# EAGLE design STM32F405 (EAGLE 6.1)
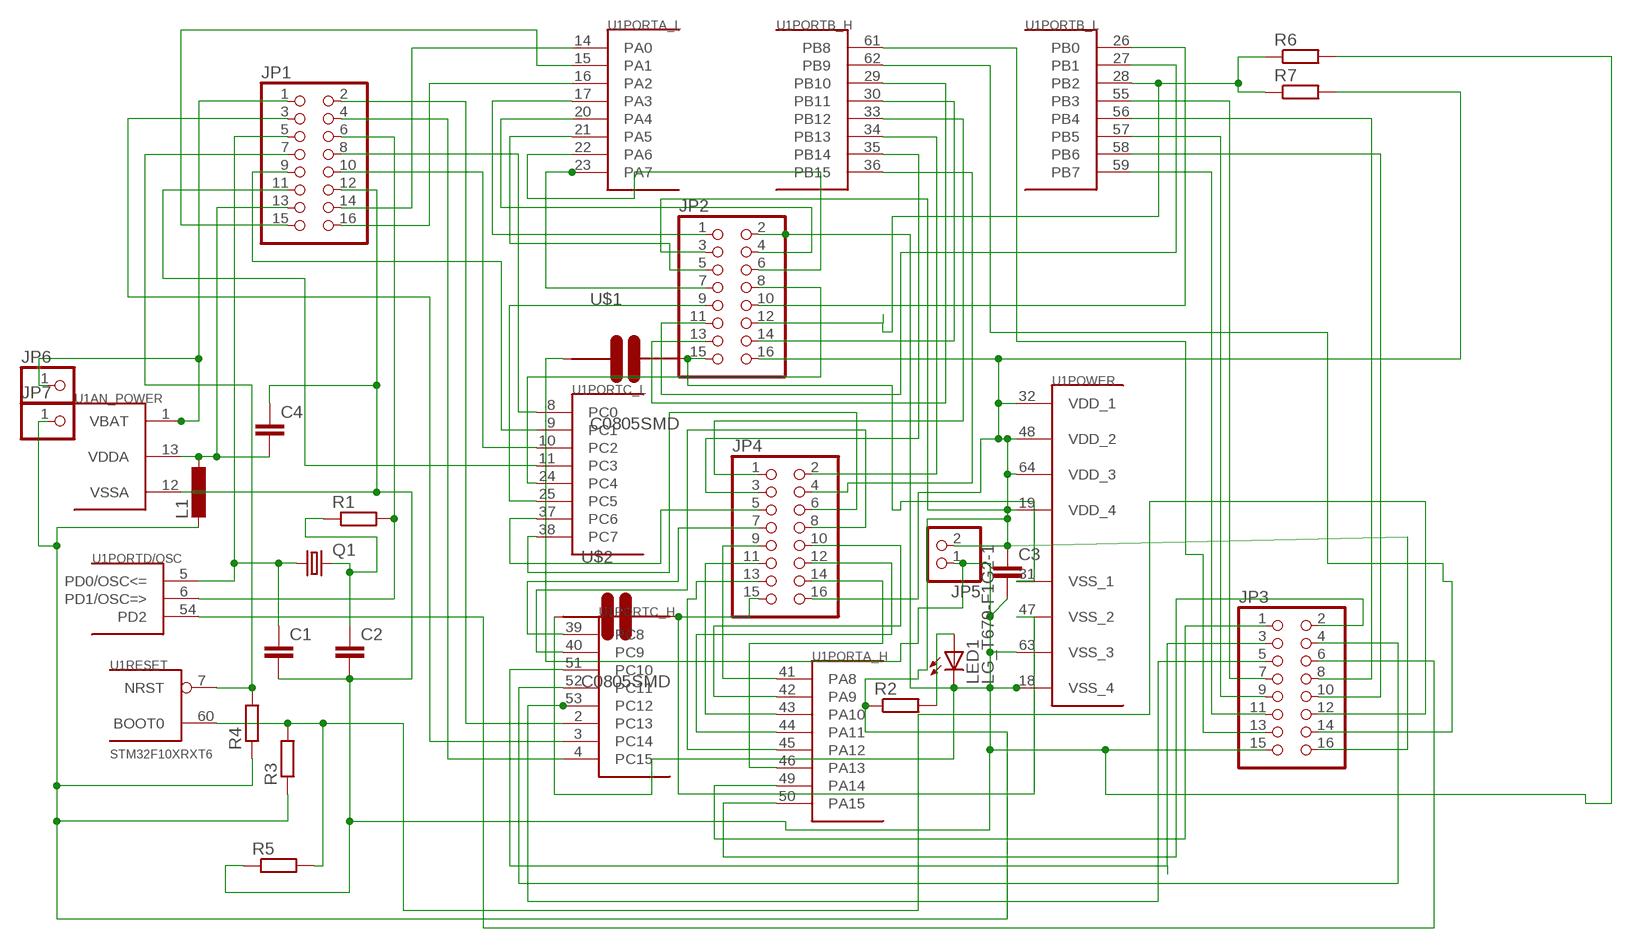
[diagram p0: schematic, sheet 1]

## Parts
C1  C-EUC0805  [C0805]
C2  C-EUC0805  [C0805]
C3  C-EUC1206  [C1206]
C4  C-EUC0805  [C0805]
JP1  PINHD-2X8  [2X08]
JP2  PINHD-2X8  [2X08]
JP3  PINHD-2X8  [2X08]
JP4  PINHD-2X8  [2X08]
JP5  PINHD-1X2  [1X02]
JP6  PINHD-1X1  [1X01]
JP7  PINHD-1X1  [1X01]
L1  L-EUL1812  [L1812]
LED1  LG_T679-F1G2-1  [PLCC2]
Q1  CRYSTALHC49S  [HC49/S]
R1  R-EU_R0805  [R0805]
R2  R-EU_R0805  [R0805]
R3  R-EU_R0805  [R0805]
R4  R-EU_R0805  [R0805]
R5  R-EU_R0805  [R0805]
R6  R-EU_M0805  [M0805]
R7  R-EU_M0805  [M0805]
U1  STM32F10XRXT6  [TQFP64]
U$1  C0805SMD  [C0805]
U$2  C0805SMD  [C0805]

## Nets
N$1: JP2.8 U1.24(PORTC_L:PC4)
N$2: C3.1 JP2.3 JP2.16 JP3.16 JP4.16 JP5.2 JP7.1 L1.2 R2.1 R3.1 R4.1 R7.2 U1.19(POWER:VDD_4) U1.32(POWER:VDD_1) U1.48(POWER:VDD_2) U1.64(POWER:VDD_3)
N$3: C4.2 JP1.13 L1.1 U1.13(AN_POWER:VDDA)
N$6: JP1.6 R1.2 U1.6(PORTD/OSC:PD1/OSC=>)
N$7: JP1.7 R4.2 U1.7(RESET:NRST)
N$8: JP1.14 U1.14(PORTA_L:PA0)
N$9: JP1.16 U1.16(PORTA_L:PA2)
N$10: JP1.15 U1.15(PORTA_L:PA1)
N$11: JP1.8 U1.8(PORTC_L:PC0)
N$12: JP1.9 U1.9(PORTC_L:PC1)
N$13: JP1.10 U1.10(PORTC_L:PC2)
N$14: JP1.11 U1.11(PORTC_L:PC3)
N$15: JP1.2 U1.2(PORTC_H:PC13)
N$16: JP1.4 U1.4(PORTC_H:PC15)
N$17: JP1.3 U1.3(PORTC_H:PC14)
N$18: JP2.1 U1.17(PORTA_L:PA3)
N$21: JP2.4 U1.20(PORTA_L:PA4)
N$22: JP2.5 U1.21(PORTA_L:PA5)
N$23: JP2.7 U1.23(PORTA_L:PA7)
N$24: JP2.6 U1.22(PORTA_L:PA6)
N$25: JP2.9 U1.25(PORTC_L:PC5)
N$26: JP2.10 U1.26(PORTB_L:PB0)
N$27: JP2.11 U1.27(PORTB_L:PB1)
N$28: JP2.12 R6.1 R7.1 U1.28(PORTB_L:PB2)
N$29: JP2.13 U1.29(PORTB_H:PB10)
N$30: JP2.14 U1.30(PORTB_H:PB11)
N$33: JP4.1 U1.33(PORTB_H:PB12)
N$34: JP4.2 U1.34(PORTB_H:PB13)
N$35: JP4.3 U1.35(PORTB_H:PB14)
N$36: JP4.4 U1.36(PORTB_H:PB15)
N$37: JP4.5 U1.37(PORTC_L:PC6)
N$38: JP4.6 U1.38(PORTC_L:PC7)
N$39: JP4.7 U1.39(PORTC_H:PC8)
N$40: JP4.8 U1.40(PORTC_H:PC9)
N$41: JP4.9 U1.41(PORTA_H:PA8)
N$42: JP4.10 U1.42(PORTA_H:PA9)
N$43: JP4.11 U1.43(PORTA_H:PA10)
N$44: JP4.12 U1.44(PORTA_H:PA11)
N$45: JP4.13 U1.45(PORTA_H:PA12)
N$46: JP4.14 U1.46(PORTA_H:PA13)
N$49: JP3.1 U1.49(PORTA_H:PA14)
N$50: JP3.2 U1.50(PORTA_H:PA15)
N$51: JP3.3 U1.51(PORTC_H:PC10)
N$52: JP3.4 U1.52(PORTC_H:PC11)
N$53: JP3.5 U1.53(PORTC_H:PC12)
N$54: JP3.6 U1.54(PORTD/OSC:PD2)
N$55: JP3.7 U1.55(PORTB_L:PB3)
N$56: JP3.8 U1.56(PORTB_L:PB4)
N$57: JP3.9 U1.57(PORTB_L:PB5)
N$58: JP3.10 U1.58(PORTB_L:PB6)
N$59: JP3.11 U1.59(PORTB_L:PB7)
N$60: C1.1 JP1.5 Q1.1 U1.5(PORTD/OSC:PD0/OSC<=)
N$62: JP3.12 R3.2 R5.2 U1.60(RESET:BOOT0)
N$63: JP3.13 U1.61(PORTB_H:PB8)
N$64: JP3.14 U1.62(PORTB_H:PB9)
N$68: JP2.15 U1.31(POWER:VSS_1) U$1.2
N$126: C1.2 C2.2 C3.2 C4.1 JP1.12 JP2.2 JP3.15 JP5.1 LED1.C R5.1 R6.2 U1.12(AN_POWER:VSSA) U1.18(POWER:VSS_4) U1.63(POWER:VSS_3) U$1.1 U$2.1
N$129: LED1.A R2.2
N$133: JP1.1 JP6.1 U1.1(AN_POWER:VBAT)
N$223: C2.1 Q1.2 R1.1
N$231: JP4.15 U1.47(POWER:VSS_2) U$2.2

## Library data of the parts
C1-C4 = rcl:C-EU: CAPACITOR, European symbol
JP1-JP4 = pinhead:PINHD-2X8: PIN HEADER
JP5 = pinhead:PINHD-1X2: PIN HEADER
JP6 JP7 = pinhead:PINHD-1X1: PIN HEADER
L1 = rcl:L-EU: INDUCTOR, European symbol
LED1 = led:*_T679-?-1: LC TOPLED® Low Current LED; COLOR: green
Q1 = crystal:CRYSTAL: CRYSTAL
R1-R7 = rcl:R-EU_: RESISTOR, European symbol
U1 = stm32:STM32F10XRXT6: STM32F101/103 64pin LQFP
U$1 U$2 = cansat_jecnaci:C0805SMD: kondenzator v provedeni SMD0805

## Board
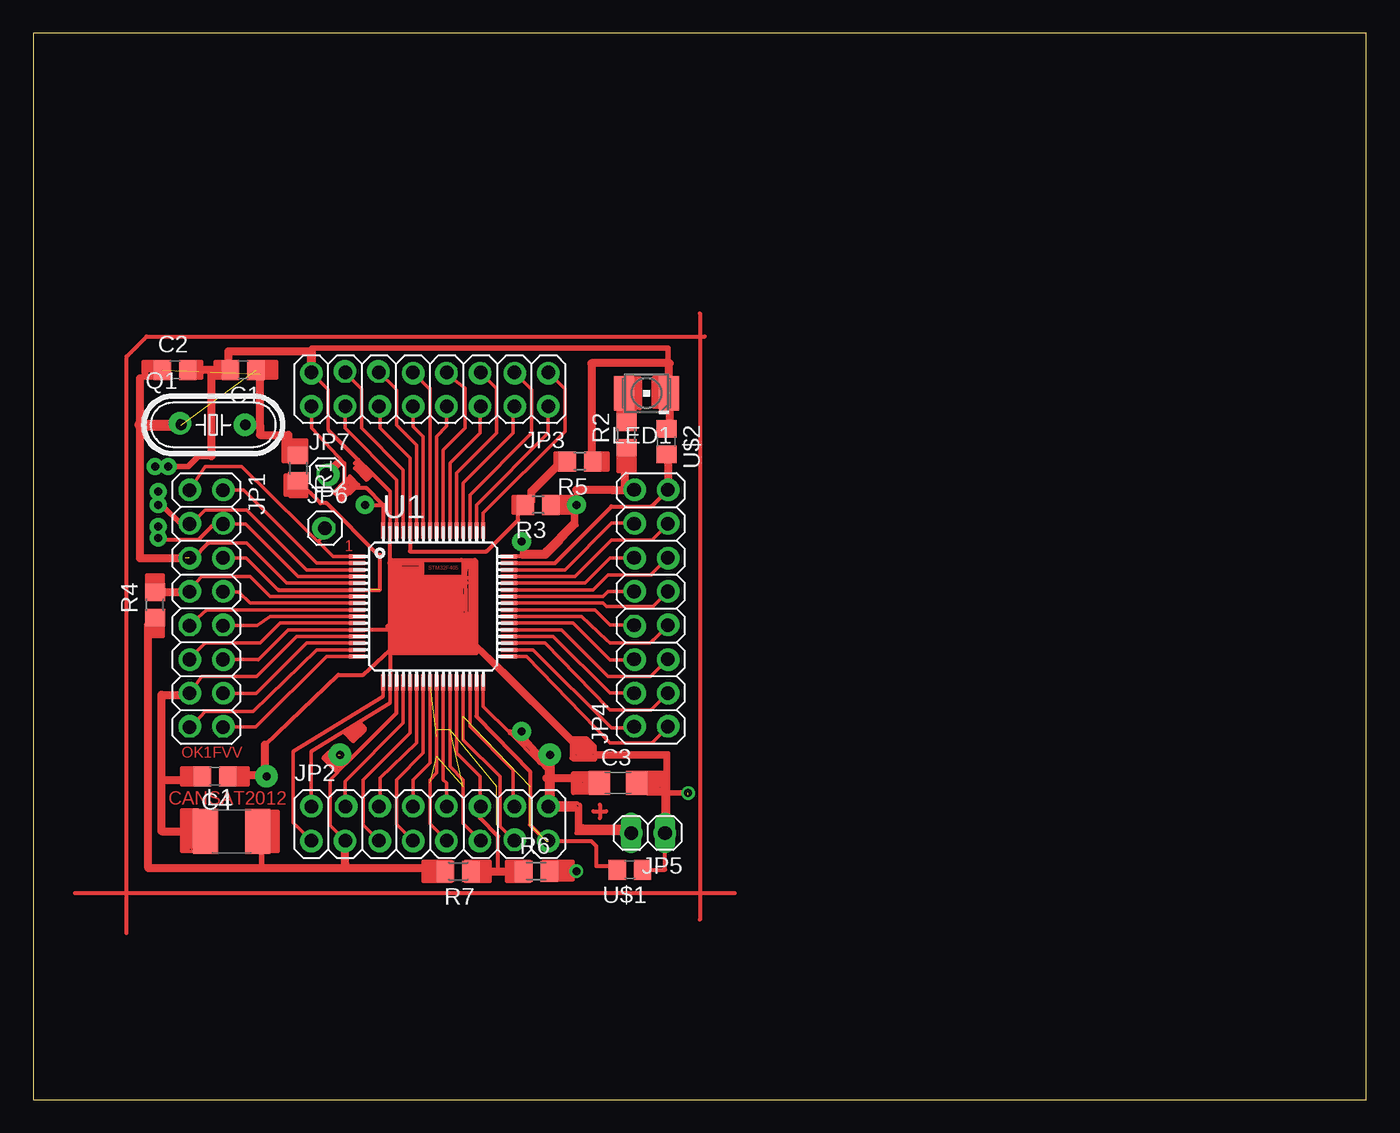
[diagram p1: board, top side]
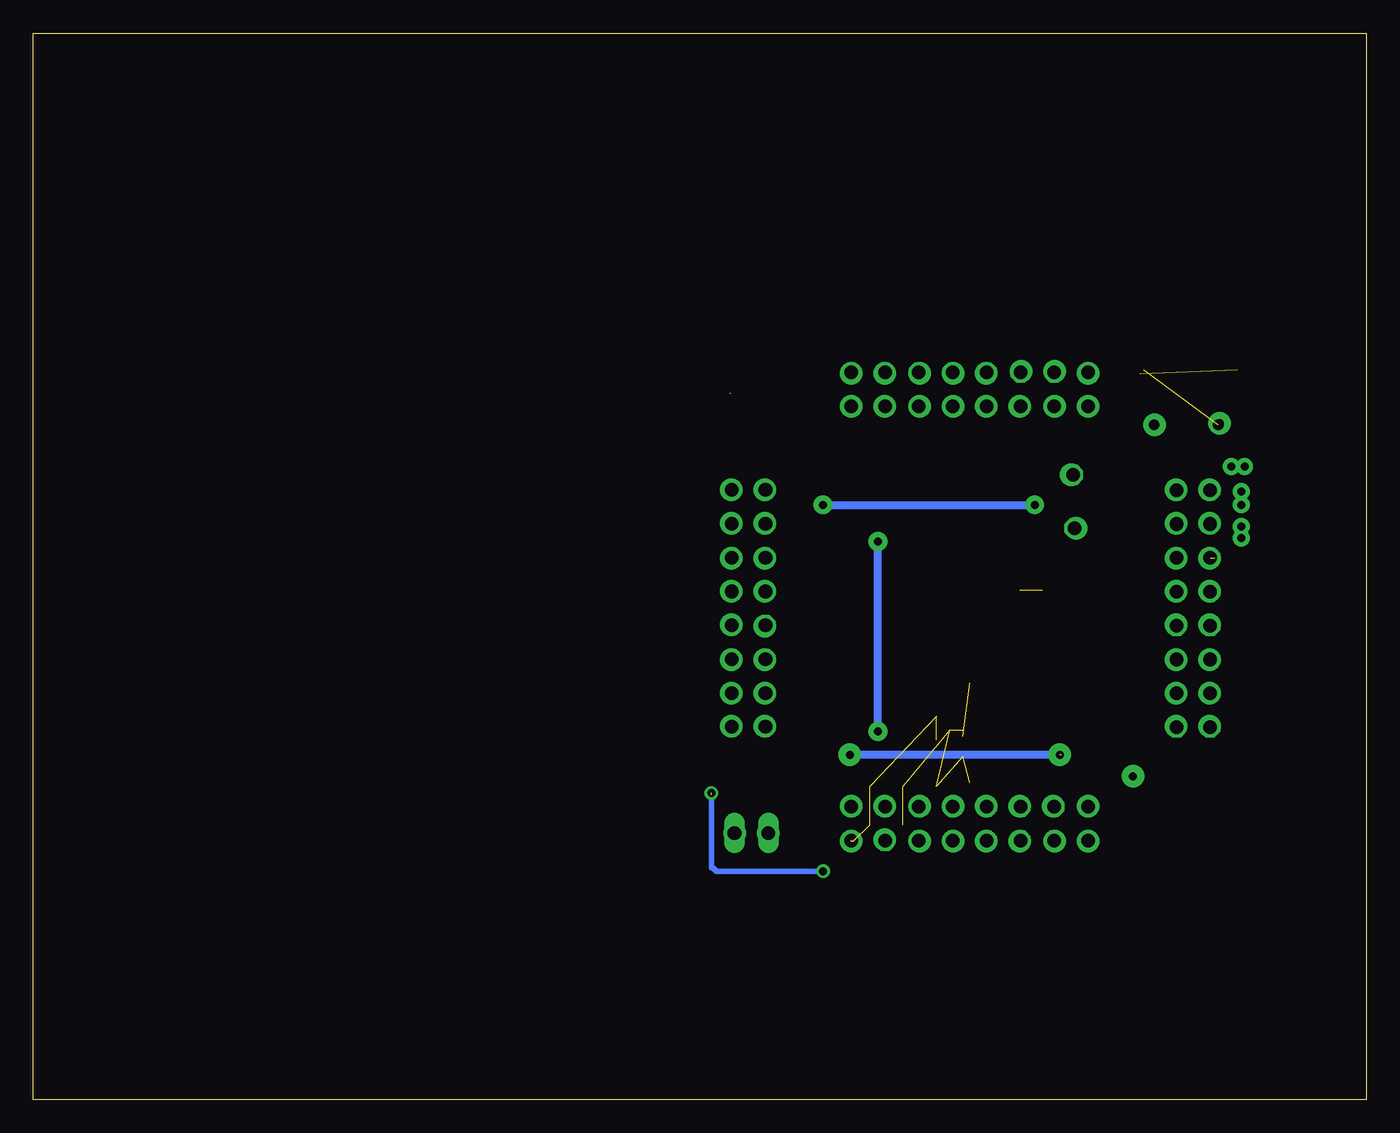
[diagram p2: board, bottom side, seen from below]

Size 100 x 80 mm. Coordinates in mm from the lower left corner, seen from the top.
Outline: 0,0 100,0 100,80 0,80 0,0
Copper layers (1*16): Top 0.035mm / dielectric 1.5mm / Bottom 0.035mm
Design rules: minimum track width 10mil, minimum drill 24mil, track to track 8mil, track to pad 8mil, pad to pad 8mil, via to via 8mil, smd to smd 8mil, copper to edge 40mil, drill to drill 8mil, minimum pad ring 10mil, minimum via ring 8mil, stop-mask expansion 4mil, vias tented up to drill 0mil, thermal gap 10mil

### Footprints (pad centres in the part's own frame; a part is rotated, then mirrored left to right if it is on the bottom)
C0805 = smd 1.3 x 1.5: 1 -0.95,0; 2 0.95,0
C1206 = smd 1.6 x 1.8: 1 -1.4,0; 2 1.4,0
2X08 = drill 1.016 octagon: 1 -8.89,-1.27; 2 -8.89,1.27; 3 -6.35,-1.27; 4 -6.35,1.27; 5 -3.81,-1.27; 6 -3.81,1.27; 7 -1.27,-1.27; 8 -1.27,1.27; 9 1.27,-1.27; 10 1.27,1.27; 11 3.81,-1.27; 12 3.81,1.27; 13 6.35,-1.27; 14 6.35,1.27; 15 8.89,-1.27; 16 8.89,1.27
1X02 = drill 1.016 long: 1 -1.27,0; 2 1.27,0
1X01 = drill 1.016 octagon: 1 0,0
L1812 = smd 1.9 x 3.4: 1 -1.95,0; 2 1.95,0
PLCC2 = smd 2.6 x 1.5: A 0,1.7; C 0,-1.7
HC49/S = drill 0.813: 1 -2.413,0; 2 2.413,0
R0805 = smd 1.3 x 1.5: 1 -0.95,0; 2 0.95,0
M0805 = smd 1.3 x 1.6: 1 -0.95,0; 2 0.95,0
TQFP64 = smd 1.2 x 0.3: 1 -5.7,3.75; 2 -5.7,3.25; 3 -5.7,2.75; 4 -5.7,2.25; 5 -5.7,1.75; 6 -5.7,1.25; 7 -5.7,0.75; 8 -5.7,0.25; 9 -5.7,-0.25; 10 -5.7,-0.75; 11 -5.7,-1.25; 12 -5.7,-1.75; 13 -5.7,-2.25; 14 -5.7,-2.75; 15 -5.7,-3.25; 16 -5.7,-3.75; 33 5.7,-3.75; 34 5.7,-3.25; 35 5.7,-2.75; 36 5.7,-2.25; 37 5.7,-1.75; 38 5.7,-1.25; 39 5.7,-0.75; 40 5.7,-0.25; 41 5.7,0.25; 42 5.7,0.75; 43 5.7,1.25; 44 5.7,1.75; 45 5.7,2.25; 46 5.7,2.75; 47 5.7,3.25; 48 5.7,3.75 | smd 0.3 x 1.2: 17 -3.75,-5.7; 18 -3.25,-5.7; 19 -2.75,-5.7; 20 -2.25,-5.7; 21 -1.75,-5.7; 22 -1.25,-5.7; 23 -0.75,-5.7; 24 -0.25,-5.7; 25 0.25,-5.7; 26 0.75,-5.7; 27 1.25,-5.7; 28 1.75,-5.7; 29 2.25,-5.7; 30 2.75,-5.7; 31 3.25,-5.7; 32 3.75,-5.7; 49 3.75,5.7; 50 3.25,5.7; 51 2.75,5.7; 52 2.25,5.7; 53 1.75,5.7; 54 1.25,5.7; 55 0.75,5.7; 56 0.25,5.7; 57 -0.25,5.7; 58 -0.75,5.7; 59 -1.25,5.7; 60 -1.75,5.7; 61 -2.25,5.7; 62 -2.75,5.7; 63 -3.25,5.7; 64 -3.75,5.7

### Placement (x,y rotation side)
C1  15.75,54.75 180 top
C2  10.62,54.75 0 top
C3  43.88,23.75 0 top
C4  13.62,24.25 180 top
JP1  12.97,36.83 270 top
JP2  29.75,20.69 0 top
JP3  29.75,53.28 180 top
JP4  46.34,36.85 90 top
JP5  46.12,20 180 top
JP6  21.88,42.88 0 top
JP7  22,46.88 0 top
L1  14.88,20.12 0 top
LED1  46,53 90 top
Q1  13.5,50.62 0 top
R1  19.88,47.38 270 top
R2  44.5,49.88 90 top
R3  37.88,44.62 180 top
R4  9.12,37.12 90 top
R5  41,47.88 180 top
R6  37.75,17.12 0 top
R7  31.88,17.12 180 top
U1  30,37 0 top
U$1  44.75,17.25 180 top
U$2  47.5,49.38 270 top

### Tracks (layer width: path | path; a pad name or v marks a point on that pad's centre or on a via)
N$1  (via drill 0.7 pad 1.68)  (1 unrouted)
  Top 0.254: JP2.8 28.48,21.98 v28.5,22 28.5,24 29.75,25.25 U1.24 | 29.75,23.25 29.75,24 30.25,24.5 30.25,27.25
N$2  (via drill 0.6 pad 1.42, 0.6 pad 1.68)  (1 unrouted)
  Top 0.254: JP2.16 38.5,22.1 38.5,24.12 38.5,24.75 38,25.25 37.94,25.31 35.75,27.5 33.75,29.5 33.75,31.12 | JP4.16 44.38,45.75 | 40.78,43.09 40.48,42.78 38.5,40.75 | 43.39,45.74 43.5,45.75 | JP3.16 20.88,51.99 20.88,50.38 23.35,47.72 22.85,47.72 | JP2.3 22.25,20.57 22.25,24 23.5,25.25 | 29.5,17.38 29.5,16.75 | 29.5,16.75 29.5,16.62 | 29.5,16.75 29.62,16.75 | 30.38,16.62 30.38,16.75 29.62,16.75 | 29.62,17.38 29.62,16.88 | 29.62,16.75 29.62,16.88 | 29.62,16.88 29.88,16.88 29.88,17.38 | 30.12,17.38 30,17.38 30,16.88 | 30,16.88 30.12,16.88 | 30.12,16.88 30.25,16.88 | 30.25,17.25 30.12,17.25 30.12,16.88 | 30,16.88 29.25,16.88 29.25,16.38 30.25,16.38 | 30.25,16.38 31.38,16.38 | 30.25,16.38 30.25,17.12
  Top 0.305: 26.25,44.62 U1.64 26.25,42.5 | 36.62,40.75 38.5,40.75 39.62,41.88 | 36.62,40.75 U1.48 | 40.78,43.09 40.75,43.12 v40.75,44.62 R3.1 | v24.88,44.62 26.25,44.62 | 33.75,31.12 U1.32 | v36.62,41.88 36.62,40.75 | v36.62,27.62 35.75,27.62 35.75,27.5 | U1.19 27.25,29 23.5,25.25 22.88,25.88 | 37.94,25.31 38,25.38 38,25.25 38.62,25.88 v38.75,25.88 | JP5.2 40.75,20 40.75,21.75 | 40.75,21.75 40.75,21.88 40.66,21.96 JP2.16 | 42.1,24.12 C3.1 | 17.12,19.82 L1.2 | 23.38,17.38 23.4,17.65 | 8.62,35.67 R4.1 | 44.38,48.8 R2.1 | 40.75,21.75 39.25,21.75 | R7.2 30.68,17.38 30.12,17.38 29.88,17.38 29.62,17.38 29.5,17.38 | 43.39,45.74 43.15,45.75 | 26.25,44.62 25,45.88 24.12,45.88 23.75,45.5 23.12,46.12 | 23.12,46.12 23.35,46.35 23.35,47.72 | 23.12,46.12 23,46 | 23,46 22.62,45.62 22.62,45.5 23.12,45 23.75,45.62 | 23,46 23.38,45.62 | 23.5,45.5 23.38,45.62 | 23.38,45.62 22.88,45.62 23.12,45.38 23.12,45.12 23.38,45.38 23.38,45.5
  Top 0.406: 17.12,17.38 17.12,19.82 | 40.75,45.75 v40.75,44.62
  Top 0.61: 43.38,45.75 43.5,45.75 44.38,45.75 44.38,48.8 | 38.5,24.12 42.1,24.12 | 23.4,17.65 JP2.3 | 8.62,35.67 8.62,17.38 17.12,17.38 23.38,17.38 29.5,17.38 | 22.85,47.72 JP7.1 | 43.15,45.75 40.75,45.75
  Bottom 0.61: v40.75,44.62 v24.88,44.62 | v36.62,27.62 v36.62,41.88 | v23,25.88 v38.75,25.88
N$3  (via drill 0.7 pad 1.68)
  Top 0.254: U1.13 19.75,34.75 16.75,31.75 12.62,31.75 v11.75,30.5 11.61,30.48 JP1.13
  Top 0.305: 11.5,30.38 11.61,30.48 | 12.43,24 C4.2
  Top 0.61: 11.5,30.38 9.62,30.38 9.62,24 | 9.62,24 9.62,20.12 L1.1 | 9.62,24 12.43,24
N$4
  Top 0.305: 41.88,23 40.5,23 40.5,24.5 41.75,24.5 41.62,24.38 40.88,24.25 40.62,24.25 40.75,23.25 41.62,23.25 41.62,24 40.88,23.88 41,23.38 41.38,23.5 41.38,23.75 41.12,23.62
N$5  (via drill 0.6 pad 1.68)
  other vias: 44.88,20
N$6  (1 unrouted)
  Top 0.254: 18.38,38.25 15.98,40.64 JP1.6
  Top 0.305: 18.38,38.25 26,38.25 26,40.88 25.88,40.88 22,44.75 21.55,44.75 R1.2
N$7
  Top 0.254: U1.7 17.75,37.75 16.25,39.25 12.62,39.25 11.57,38.08 JP1.7
  Top 0.305: R4.2 9.15,38.1
  Top 0.61: 9.15,38.1 JP1.7
N$8
  Top 0.254: U1.14 20.5,34.25 16.73,30.48 JP1.14
N$9
  Top 0.254: U1.16 22,33.25 16.69,27.94 JP1.16
N$10
  Top 0.254: U1.15 21.25,33.75 16.5,29.12 12.88,29.12 11.82,27.95 JP1.15
N$11
  Top 0.254: U1.8 16.25,37.25 15.4,38.1 JP1.8
N$12
  Top 0.254: U1.9 13,36.75 11.69,35.56 JP1.9
N$13
  Top 0.254: U1.10 17.75,36.25 16.81,35.56 JP1.10
N$14
  Top 0.254: U1.11 18.5,35.75 17,34.25 12.88,34.25 11.7,33.08 JP1.11
N$15
  Top 0.254: U1.2 21.25,40.25 15.78,45.72 JP1.2
N$16
  Top 0.254: U1.4 19.88,39.25 15.95,43.18 JP1.4
N$17
  Top 0.254: U1.3 20.5,39.75 16,44.25 12.88,44.25 11.82,43.2 JP1.3
N$18
  Top 0.254: U1.17 26.25,30.25 19.5,26.12 19.5,20.75 19.75,20.5 19.78,20.5 JP2.1
N$19  (via drill 0.6 pad 1.68)
  other vias: 17.5,24.25
N$20  (via drill 0.6 pad 1.68)
  other vias: 11,50.75
N$21
  Top 0.254: U1.20 27.75,28.25 23.38,23.88 23.38,21.93 JP2.4
N$22
  Top 0.254: U1.21 28.25,27.5 24.75,24 24.75,20.61 JP2.5
N$23
  Top 0.254: U1.23 29.25,26 27.25,24 27.25,20.65 JP2.7
N$24
  Top 0.254: U1.22 28.75,26.75 26,24.12 26,22.14 JP2.6
N$25  (3 unrouted)
  Top 0.254: 30.25,25.75 U1.25 | JP2.9 29.75,20.69 29.75,23.75 | 32.25,23.5 32.25,24 31.25,25 31.25,27.75
N$26  (via drill 0.7 pad 1.68)
  Top 0.254: JP2.10 31,21.98 v31,22 31,23.75 30.75,24 U1.26
N$27  (3 unrouted)
  Top 0.254: 31.25,27.75 U1.27 | JP2.11 32.25,20.73 32.25,23.5
N$28
  Top 0.254: JP2.12 33.5,22.02 33.5,24.25 31.75,26 U1.28
  Top 0.305: 33.5,22.02 33.5,21.12 34.88,19.75 34.88,17.12
  Top 0.61: R6.1 34.88,17.12 R7.1
N$29  (3 unrouted)
  Top 0.254: JP2.13 35.02,20.5 35,20.5 35,24.25 32.25,27 U1.29
N$30
  Top 0.254: JP2.14 36,22.06 36,24.75 32.75,28 U1.30
N$31
  Top 0.305: 50.38,57.25 8.5,57.25 7,55.75 7,12.5
N$32  (via drill 0.6 pad 1.68)
  other vias: 15.88,50.62
N$33
  Top 0.254: JP4.1 46.4,26.75 43.25,26.75 37,33.25 U1.33
N$34
  Top 0.254: JP4.2 44.91,27.88 43.38,27.88 37.5,33.75 U1.34
N$35
  Top 0.254: JP4.3 46.36,29.25 43.25,29.25 43.12,29.38 38.38,34.25 U1.35
N$36
  Top 0.254: JP4.4 43.25,30.5 39,34.75 U1.36
N$37
  Top 0.254: JP4.5 46.32,31.75 43.12,31.75 39.62,35.25 U1.37
N$38
  Top 0.254: JP4.6 45.03,33 43.25,33 40.5,35.75 U1.38
N$39
  Top 0.254: JP4.7 46.53,34.5 46.5,34.5 46.25,34.25 43.25,34.25 43,34.5 41.12,36.25 U1.39
N$40
  Top 0.254: JP4.8 44.87,35.62 43.25,35.62 42.12,36.75 U1.40
N$41
  Top 0.254: JP4.9 46.49,37 43,37 42.75,37.25 U1.41
N$42
  Top 0.254: JP4.10 44.94,38.12 43.12,38.12 42.75,37.75 U1.42
N$43
  Top 0.254: JP4.11 46.38,39.42 46.38,39.38 43.12,39.38 42,38.25 U1.43
N$44
  Top 0.254: JP4.12 45.03,40.62 43.38,40.62 43.25,40.62 41.38,38.75 U1.44
N$45
  Top 0.254: JP4.13 46.41,42 43.38,42 40.62,39.25 U1.45
N$46
  Top 0.254: JP4.14 45.02,43.25 43.38,43.25 39.88,39.75 U1.46
N$47
  Top 0.254: 8.38,55.25 8.5,55.25 8.5,54.38
N$48  (via drill 0.6 pad 1.68)
  other vias: 47.38,20
N$49
  Top 0.254: JP3.1 39.88,53.31 39.88,50.12 33.75,44 U1.49
N$50
  Top 0.254: JP3.2 38.62,51.99 38.62,50 33.25,44.62 U1.50
N$51
  Top 0.254: JP3.3 37.38,53.27 37.38,50 32.75,45.38 U1.51
N$52
  Top 0.254: JP3.4 36,51.91 36,50 32.25,46.25 U1.52
N$53
  Top 0.254: JP3.5 34.75,53.36 34.75,50 31.75,47 U1.53
N$54
  Top 0.254: JP3.6 33.5,51.95 33.5,50 31.25,47.75 U1.54
N$55
  Top 0.254: U1.55 30.75,48.75 32.38,50.38 32.38,53.38 31.2,54.3 JP3.7
N$56
  Top 0.254: U1.56 30.25,49.75 31.02,50.52 JP3.8
N$57
  Top 0.254: JP3.9 29.66,53.38 29.75,53.38 U1.57
N$58
  Top 0.254: JP3.10 28.5,51.99 28.5,50.5 29.25,49.75 U1.58
N$59
  Top 0.254: JP3.11 27.12,53.37 27.25,53.25 27.25,50.62 28.75,49.12 U1.59
N$60  (2 unrouted)
  Top 0.254: U1.5 19,38.75 16,41.75 13.12,41.75 | 11.7,40.58 JP1.5
  Top 0.305: Q1.1 11,50.54 | 11.38,40.62 8,40.62 8,50.62 | 13.12,41.75 12.02,40.64 JP1.5
  Top 0.813: 8,50.62 Q1.1
N$61
  Top 0.305: 39.12,22.25 40.75,22.25 41,22.12 41,20.25 | 41,20.12 41,20.25 | 41,20.25 44.12,20.25 44.25,20.12 41.25,20.5 44.25,20.5
N$62
  Top 0.254: JP3.12 26,51.95 26,50.38 28.25,48.12 U1.60
  Top 0.305: U1.60 28.25,41.12 34,41.12 36.38,43.5 36.38,44 36.92,44.55 | 36.92,44.55 R3.2 | 36.92,44.55 37,44.62 37.12,44.62 37.38,44.88 | 39.62,47.88 R5.2
  Top 0.61: 37.38,44.88 37.38,45.62 39.62,47.88
N$63
  Top 0.254: JP3.13 24.62,53.33 24.62,50.38 27.75,47.25 U1.61
N$64
  Top 0.254: JP3.14 23.38,51.98 23.38,50.38 27.25,46.5 U1.62
N$65  (via drill 0.7 pad 1.68)
  other vias: 11.75,45.75
N$66  (via drill 0.7 pad 1.68)
  other vias: 14.25,45.75
N$67  (via drill 0.7 pad 1.68)
  other vias: 14.25,43.25
N$68  (3 unrouted)
  Top 0.305: U1.31 33.25,28.75 37.25,24.62 37.25,20.62 38.5,19.38 38.62,19.38 41.88,19.38 42.25,19 42.25,17.5 43.55,17.5 U$1.2
N$69  (via drill 0.7 pad 1.68)
  other vias: 14.25,40.62
N$70  (via drill 0.7 pad 1.68)
  other vias: 14.25,38.12
N$71  (via drill 0.7 pad 1.68)
  other vias: 14.25,35.62
N$72  (via drill 0.7 pad 1.68)
  other vias: 11.75,35.62
N$73  (via drill 0.7 pad 1.68)
  other vias: 11.75,38.12
N$74  (via drill 0.7 pad 1.68)
  other vias: 11.75,40.62
N$75  (via drill 0.7 pad 1.68)
  other vias: 14.25,33
N$76  (via drill 0.7 pad 1.68)
  other vias: 14.25,30.5
N$77  (via drill 0.7 pad 1.68)
  other vias: 14.25,28
N$78  (via drill 0.7 pad 1.68)
  other vias: 11.75,28
N$79  (via drill 0.7 pad 1.68)
  other vias: 11.75,33
N$80  (via drill 0.7 pad 1.68)
  other vias: 20.88,22
N$81  (via drill 0.7 pad 1.68)
  other vias: 23.5,22
N$82  (via drill 0.7 pad 1.68)
  other vias: 26,22
N$83  (via drill 0.7 pad 1.68)
  other vias: 31,19.38
N$84  (via drill 0.7 pad 1.68)
  other vias: 28.5,19.38
N$85  (via drill 0.7 pad 1.68)
  other vias: 26,19.38
N$86  (via drill 0.7 pad 1.68)
  other vias: 23.38,19.38
N$87  (via drill 0.7 pad 1.68)
  other vias: 20.88,19.38
N$88  (via drill 0.7 pad 1.68)
  other vias: 33.5,22
N$89  (via drill 0.7 pad 1.68)
  other vias: 36.12,22
N$90  (via drill 0.7 pad 1.68)
  other vias: 38.62,22
N$91  (via drill 0.7 pad 1.68)
  other vias: 38.62,19.38
N$92  (via drill 0.7 pad 1.68)
  other vias: 36.12,19.5
N$93  (via drill 0.7 pad 1.68)
  other vias: 33.5,19.38
N$94  (via drill 0.7 pad 1.68)
  other vias: 45.12,28
N$95  (via drill 0.7 pad 1.68)
  other vias: 47.62,28
N$96  (via drill 0.7 pad 1.68)
  other vias: 47.62,30.5
N$97  (via drill 0.7 pad 1.68)
  other vias: 47.62,33
N$98  (via drill 0.7 pad 1.68)
  other vias: 47.62,35.62
N$99  (via drill 0.7 pad 1.68)
  other vias: 47.62,38.12
N$100  (via drill 0.7 pad 1.68)
  other vias: 45.12,30.5
N$101  (via drill 0.7 pad 1.68)
  other vias: 45.12,33
N$102  (via drill 0.7 pad 1.68)
  other vias: 45.12,35.5
N$103  (via drill 0.7 pad 1.68)
  other vias: 45.12,38.12
N$104  (via drill 0.7 pad 1.68)
  other vias: 47.62,40.62
N$105  (via drill 0.7 pad 1.68)
  other vias: 45.12,40.62
N$106  (via drill 0.7 pad 1.68)
  other vias: 45.12,43.25
N$107  (via drill 0.7 pad 1.68)
  other vias: 47.62,43.25
N$108  (via drill 0.7 pad 1.68)
  other vias: 47.62,45.75
N$109  (via drill 0.7 pad 1.68)
  other vias: 45.12,45.75
N$110  (via drill 0.7 pad 1.68)
  other vias: 38.62,52
N$111  (via drill 0.7 pad 1.68)
  other vias: 38.62,54.5
N$112  (via drill 0.7 pad 1.68)
  other vias: 36.12,52
N$113  (via drill 0.7 pad 1.68)
  other vias: 36.12,54.5
N$114  (via drill 0.7 pad 1.68)
  other vias: 33.5,52
N$115  (via drill 0.7 pad 1.68)
  other vias: 33.5,54.5
N$116  (via drill 0.7 pad 1.68)
  other vias: 31,54.5
N$117  (via drill 0.7 pad 1.68)
  other vias: 31,52
N$118  (via drill 0.7 pad 1.68)
  other vias: 28.5,52
N$119  (via drill 0.7 pad 1.68)
  other vias: 28.5,54.5
N$120  (via drill 0.7 pad 1.68)
  other vias: 25.88,54.62
N$121  (via drill 0.7 pad 1.68)
  other vias: 26,52
N$122  (via drill 0.7 pad 1.68)
  other vias: 23.38,52
N$123  (via drill 0.7 pad 1.68)
  other vias: 23.38,54.62
N$124  (via drill 0.7 pad 1.68)
  other vias: 20.88,52
N$125  (via drill 0.7 pad 1.68)
  other vias: 20.88,54.5
N$126  (via drill 0.6)  (2 unrouted)
  Top 0.254: JP3.15 22.12,53.28 22.12,50.25 | U1.63 26.75,45.62 | U1.18 26.75,29.75 20.86,26.11 JP2.2 | U1.12 19.12,35.25 16.88,33 16.86,33.02 JP1.12
  Top 0.305: 47.62,21.12 47.62,26 42.12,26 | 40.5,25.5 42.12,25.5 42.12,26 | 42.12,26 42.12,26.5 41.5,27.12 40.38,27.12 | 40.38,27.12 40.38,25.62 40.5,25.62 | 40.5,25.62 41.25,25.62 41.25,27 40.62,26.88 40.5,25.62 | 40.5,25.62 40.88,26.75 40.88,25.75 41.12,26.62 41.5,26.88 42,26.25 41.88,26 41.38,26 41.12,26.75 41.12,25.88 41.5,26.62 41.75,26.25 41.5,26.12 | 40.38,27.12 42.12,26 | 40.38,27.12 35.5,32 33.25,34.12 | 33.25,33.75 33.25,33.5 26.75,33.5 | 33.25,33.75 33.25,34.12 | 33.25,34.12 33.25,40.38 | 26.75,33.5 U1.18 | 26.75,33.75 26.75,33.5 | 26.75,33.75 26.75,35.25 | 26.75,35.25 26.75,39.25 | 26.75,39.25 26.75,40.25 U1.63 | 26.75,39.25 26.88,39.25 | 26.88,39.25 27,39.25 | 27,39.25 27,33.75 33,33.75 33,39.88 | 33,39.88 33,40.12 | 33,39.88 32.75,39.88 | 32.75,39.88 32.75,40.12 | 32.75,39.88 32.75,33.88 32.5,33.88 | 32.38,39.25 32.5,34 | 32.38,39.25 32.5,40.12 | 27,39.25 32.38,39.25 | 26.88,39.25 26.88,40.5 32.12,40.5 | 27,39.62 26.88,39.25 | 27,39.25 27,39.62 | 27,39.62 27.25,39.62 27.38,38.75 | 27.25,39 32.38,39 32.5,38.75 27.38,38.75 | 27.38,38.75 27.25,39 | 27.25,39 27.25,34 | 27.25,34 27.25,33.88 | 32.5,34 27.25,34 | 32.5,34 32.5,33.88 | 32.5,33.88 32.25,33.88 32.25,34.38 | 32.25,34.5 32.12,38.62 | 32.12,38.62 32.25,39.38 32.25,40.38 32.12,40.5 | 32,38.62 27.38,38.62 | 27.38,38.62 27.38,39.25 | 27.38,38.62 27.5,34.12 27.75,34.12 27.75,38.12 | 27.75,38.38 27.75,39.12 28,39.12 28,34.12 28.25,34.12 28.25,38.75 | 28.25,38.75 28.25,39 32,39 32,38.62 | 32.12,38.62 32,38.62 | 32.12,38.62 32.12,38.75 28.38,38.75 | 28.38,38.75 28.25,38.75 | 28.38,38.5 28.38,38.75 | 28.38,38.5 28.38,34.25 | 28.38,34.25 28.38,34.12 | 28.38,34.25 31.38,34.25 | 31.62,34.25 32,34.25 32,38.5 31.62,38.5
  Top 0.305: 28.62,38.5 31.62,38.5 | 28.62,38.5 28.38,38.5 | 28.62,34.5 28.62,38.5 | 28.62,34.5 28.62,34.38 | 32.25,34.5 28.62,34.5 | 32.25,34.38 32.25,34.5 | 32.25,34.38 31.88,34.38 | 31.88,34.38 31.75,34.38 | 31.88,34.38 31.88,38.25 | 31.62,38.5 31.62,34.25 | 31.62,34.25 31.38,34.25 | 31.38,34.25 31.38,38.25 28.88,38.25 | 28.88,38.25 28.75,38.25 | 28.88,38.25 28.88,34.75 29.62,34.75 | 30.12,34.75 29.88,34.75 | 30.38,34.75 31.12,34.75 | 31.12,34.75 31.75,34.75 | 31.12,34.75 31.12,38.38 30.88,38.38 30.88,34.88 30.62,34.88 30.62,38.12 30.38,38.12 | 29.12,38.12 30.38,38.12 | 29.12,38.12 29.12,36.5 29.12,34.88 29.38,34.88 29.38,38 29.62,38 29.62,35.5 29.62,34.75 | 29.62,34.75 29.88,34.75 | 29.88,34.75 29.88,38 30.12,38 30.12,34.75 | 30.38,34.75 30.12,34.75 | 30.38,38.12 30.38,34.75 | 27.75,38.12 29.12,38.12 | 27.75,38.12 27.75,38.38 | 27.75,38.38 26.88,38.38 26.88,39.25 | 32.12,40.5 33.12,40.5 33.12,39.12 29.25,39.12 | 26.75,33.75 24.75,31.88 22.88,31.88 17.38,26.62 | 14.62,54.92 C1.2 | 20.86,56.11 20.88,56.12 | 26.75,35.25 U1.12 | 47.38,20.02 JP5.1 47.4,17.25 U$1.1 | 47.38,24.5 47.38,25.75 41.38,25.75 33.38,33.75 33.25,33.75 | 47.38,23.75 47.38,23 46.12,23 46.12,24.38 47.25,24.38 46.5,24.12 47.25,24.12 47.12,23.25 46.25,23.25 46.5,24 47.12,23.88 46.88,23.5 46.25,23.5 | 47.38,23.75 C3.2 | 47.38,24.5 45.88,24.5 | 47.38,24.5 47.38,23.75 | C4.1 14.7,24.38 | 41.88,47.95 R5.1 | 47.7,55.2 47.75,55.25 | U$2.1 47.75,50.58 | 22.12,50.25 24.38,48 | 24.38,48 24.12,47.75 24.88,47 | 24.88,47 25,47 25,47.12 25.25,47.12 | 26.75,45.62 25.38,47 | 25.38,47 25.25,47.12 | 24.38,48 25.25,47.12 | 25.38,47 25.38,46.88 25,46.5 24.12,47.38 24.38,47.62 24.62,47.62 24.88,47.38
  Top 0.305: 24.88,47.38 25.25,47 25.38,47 | 25.38,47 25.12,46.75 25,46.75 24.88,46.88 24.75,46.88 24.88,47 | 24.88,47 24.88,47.38
  Top 0.406: R6.2 v40.75,17.12 | 46.12,23 v49.12,23 | 26.75,40.25 29.12,40.25 29.12,36.5 29.62,36.5 29.62,35.5 | 29.62,35.5 32.38,35.5 | 29.62,35.5 26.62,35.5 26.62,35.38 | LED1.C 47.62,53 47.62,56.38 20.88,56.38 20.88,56.12 21,56.12 21,54.38
  Top 0.61: C1.2 C2.2 | 14.62,54.92 14.62,56.12 20.88,56.12 | JP3.15 20.86,56.11 | 47.38,23 47.38,20.02 | 14.7,24.38 17.38,24.38 17.38,26.62 | 41.88,47.95 41.88,55.25 47.75,55.25 | LED1.C 47.7,55.2 | 47.75,50.58 47.75,53
  Bottom 0.406: v40.75,17.12 48.75,17.12 49,17.38 49.12,17.38 49.12,22.88
N$127
  Top 0.305: 42,21.62 43,21.62
N$128
  Top 0.305: 42.5,22.12 42.5,21.12
N$129
  Top 0.305: R2.2 44.3,51.02 LED1.A
N$130
  Top 0.305: 3.12,15.5 52.62,15.5
N$131
  Top 0.305: 44.62,50.88 44.75,50.88 44.75,51
N$132  (via drill 0.6 pad 1.27)
  other vias: 9.38,42.12
N$133
  Top 0.254: JP1.1 11.7,45.7 12.88,47.5 15.62,47.5 22.5,40.75 | 22.5,40.75 U1.1 | 22.5,40.75 21.38,41.88 21.88,42.38 JP6.1
N$134
  Top 0.305: 50,59 50,13.5
N$135
  Top 0.305: 44.75,54.12 45.5,54.12 45.5,51.88 45,51.88
N$136
  Top 0.305: 45.12,52 45.12,54
N$137
  Top 0.305: 45.25,54 45.25,52
N$138
  Top 0.305: 47.12,54.12 46.5,54.12 46.5,52 47,52
N$139
  Top 0.305: 46.75,54 46.75,52.25
N$140
  Top 0.305: 46.88,54 46.88,52.12
N$141
  Top 0.305: 38.62,22.38 38.62,25.25
N$142
  Top 0.305: 38.25,25.25 38.5,25
N$143
  Top 0.305: 38.75,22.5 38.75,25.12
N$144
  Top 0.305: 36.5,27.12 38.12,25.5
N$145
  Top 0.305: 36.88,27.12 38,25.88
N$146
  Top 0.305: 36.75,41.12 38.62,41.12
N$147
  Top 0.305: 36.75,41 38.38,41
N$148
  Top 0.305: 38.62,41.25 40.62,43.25
N$149
  Top 0.305: 38.38,41.25 40.5,43.38 | 40.5,43.38 40.62,43.5 | 40.5,43.38 40.5,44.38
N$150
  Top 0.305: 39,22.62 39,25.25
N$151
  Top 0.305: 33.25,17.62 33.25,17.75 33.12,17.75
N$152
  Top 0.254: 38.25,17.88 40.5,17.88 40.5,16.5 38.88,16.5
N$153
  Top 0.254: 33.5,17.75 34,17.75 34,16.75 34.12,16.75 34.12,16.62 33.62,16.62 | 33.5,16.62 33.62,16.62 | 33.62,16.62 33.62,17.62 33.75,17.62 | 33.88,17.62 33.75,17.62 | 33.75,17.62 33.75,16.75 33.5,16.75 33.5,17.25 33.38,17.25 33.38,17.88 | 33.38,17.88 34.25,17.88 34.25,16.5 | 33.38,17.88 32.38,17.88 32.38,16.5 33.38,16.5 | 33.38,16.5 33.38,16.75 | 33.38,16.5 34.25,16.5 | 34.25,16.5 34.25,16.38 32.38,16.38
N$154
  Top 0.254: 39.25,17.62 40.38,17.62 40.38,16.75 | 40.38,16.75 40.38,16.62 39.38,16.62 39.38,17.5 40.25,17.5 | 40.38,16.75 39.5,16.75
N$155
  Top 0.254: 36.5,17.62 35.75,17.62 | 35.62,17.62 35.75,17.62 | 35.75,17.62 35.75,17.5 | 35.75,17.5 35.75,16.62 35.62,16.62 35.62,16.75 36.25,16.75 36.25,16.88 | 36.25,16.88 36.25,17 | 35.88,16.88 36.25,16.88 | 36.25,16.88 36.38,16.88 36.38,17.5 35.88,17.5 | 35.75,17.5 35.88,17.5 | 35.88,17.5 35.88,17.25 36.25,17.25 36.25,17.88 | 36.38,17.88 36.25,17.88 | 36.25,17.88 35.5,17.88 35.5,16.5 | 37.25,17.88 36.38,17.88 | 36.38,17.88 36.38,16.5 35.5,16.5 | 35.5,16.5 35.5,16.38 37.25,16.38
N$156
  Top 0.254: 40.12,17.38 40,17.38 | 40,17.38 39.75,17.38 | 39.75,17.38 39.5,17.38 | 39.5,17.38 38.62,17.38 38.62,17.75 40.12,17.75 40.12,16.88 | 39.5,17.38 39.5,16.88 | 39.75,17.38 39.75,16.88 | 40,17.38 40,16.88
N$157
  Top 0.254: 31.38,17.88 29.25,17.88 29.25,17.75 | 29.25,17.75 29.25,16.5 31.38,16.5 | 29.25,17.75 30.38,17.75 30.38,17.62
N$158
  Top 0.254: 29.38,17.5 30.25,17.5 30.25,17.62
N$159
  Top 0.254: 17.12,21.62 18.38,21.62 18.38,18.62 17.62,18.62
N$160
  Top 0.254: 17.88,21.5 17.88,18.75
N$161
  Top 0.254: 18.12,21.5 18,21.5 18,18.75
N$162
  Top 0.254: 18.25,21.38 18.12,21.38 18.12,18.75
N$163
  Top 0.254: 12.38,21.75 11.12,21.75 11.12,18.62 12.62,18.62 12.62,18.88
N$164
  Top 0.254: 11.25,21.62 11.38,21.62 11.38,18.75
N$165
  Top 0.254: 11.5,21.62 11.62,21.62 11.62,18.75
N$166
  Top 0.254: 11.75,21.62 11.88,21.62 11.88,18.88
N$167
  Top 0.254: 14.88,24.88 16.12,24.88 16.12,23.75 | 16,23.75 15.12,23.75 15.12,23.62 16.12,23.62 16.12,23.75 | 16.12,23.75 16,23.75 | 16,23.75 16,24 | 16,24 16,24.75 15.88,24.75 15.88,24 | 15.88,24 16,24 | 15.88,24 15.25,24 | 15.25,24 15.25,23.88 | 15.25,24 15.25,24.12 15.75,24.12 15.75,24.62 | 15.75,24.75 15.75,24.62 | 15.75,24.62 15.5,24.62 | 15,24.62 15.5,24.62 | 15.5,24.62 15.5,24.25
N$168
  Top 0.254: 12.38,24.88 11.12,24.88 11.12,23.62 12.12,23.62
N$169
  Top 0.254: 11.25,23.75 12.12,23.75 12.12,23.88
N$170
  Top 0.254: 11.25,24.62 12.12,24.62
N$171
  Top 0.254: 11.25,24.5 12.12,24.5 12.12,24.38 11.25,24.38
N$172
  Top 0.254: 11.25,24.25 12,24.25
N$173
  Top 0.254: 8.5,38.5 8.5,38.62 8.88,38.62 8.88,38.12
N$174
  Top 0.254: 8.5,38.38 8.5,39.38 9.75,39.38 9.75,39.12 | 9.75,39.12 9.75,38.62 | 9.75,39.12 8.88,39.12
N$175
  Top 0.254: 9.62,38.88 8.62,38.88 8.62,39.25
N$176
  Top 0.254: 8.88,38.75 9.62,38.75 9.62,38.62 8.75,38.62 8.75,39.25
N$177
  Top 0.254: 8.5,35.62 8.5,34.75 9.75,34.75 9.75,35.5 8.88,35.5 | 8.75,35.5 8.88,35.5 | 8.88,35.5 8.88,35.38 | 8.88,35.38 8.88,35 | 8.88,34.88 8.88,35 | 8.88,35 9.62,35 9.62,35.38 | 8.88,35.38 9.5,35.38 9.5,35.12 9,35.12 9,35.25
N$178  (via drill 0.6 pad 1.27)
  other vias: 9.38,44.62
N$179
  Top 0.254: 8.88,55.25 9,55.25 9,54.38
N$180
  Top 0.254: 8.75,55.25 8.88,55.25 8.88,54.25
N$181
  Top 0.254: 17.25,55.38 18.25,55.38 18.25,54.12 17.25,54.12
N$182
  Top 0.254: 17.38,55.25 17.38,54.38
N$183
  Top 0.254: 17.62,55.25 17.62,54.25
N$184
  Top 0.254: 18,55.25 18,54.25
N$185
  Top 0.254: 17.88,55.25 17.88,54.25 17.5,54.25
N$186
  Top 0.254: 12.12,55.38 12.62,55.38 12.62,54.12 12.12,54.12
N$187
  Top 0.254: 12.25,55.25 12.25,54.38
N$188
  Top 0.254: 12.5,55.25 12.38,55.25 12.38,54.25
N$189
  Top 0.254: 14.38,55.38 13.62,55.38 13.62,54.12 14.25,54.12
N$190
  Top 0.254: 13.88,55.25 13.75,55.25 13.75,54.38 14.12,54.38 | 14.12,55.25 14.12,54.38 | 14.12,54.38 14.12,54.25
N$191
  Top 0.254: 14,55.25 13.88,55.25 13.88,54.38
N$192
  Top 0.254: 39.62,48.5 39.12,48.5 39.12,47.25 39.5,47.25
N$193
  Top 0.254: 19.5,49.38 19.5,49.25 | 19.5,49.25 19.5,48.88 | 19.5,49.25 20.12,49.25 20.12,49.12
N$194
  Top 0.254: 20.25,49.38 20.25,48.88
N$195
  Top 0.254: 20.38,49 19.62,49
N$196
  Top 0.254: 19.25,46 19.25,45.38 | 19.25,45.38 19.25,45.25 20.5,45.25 20.5,46 | 19.25,45.38 18.88,45.38 18.88,46.88 19,46.88 | 19.25,46.88 19.12,46.88 19,46.88 | 19,46.88 19,45.5
N$197
  Top 0.254: 19.38,45.75 20.25,45.75 20.25,45.38
N$198
  Top 0.254: 19.5,45.38 19.5,45.62 20.12,45.62 20.12,45.5 19.62,45.5
N$199
  Top 0.254: 46.25,24.25 46.38,24.25 46.38,23.88
N$200
  Top 0.254: 43.88,48.75 43.88,47.62 | 43.88,47.62 45.12,47.62 | 45.12,47.62 45.12,47.75 45.12,48.25 | 45.12,48.25 45.12,48.38 | 45.12,48.25 44.25,48.25 | 43.88,47.62 43.88,47.12 45.12,47.12 45.12,47.62
N$201
  Top 0.254: 45,48.12 44.12,48.12 44.12,48.25
N$202
  Top 0.254: 44,48 45,48 45,47.75
N$203
  Top 0.254: 44,47.75 44.88,47.75
N$204
  Top 0.254: 42.38,48.5 43.12,48.5 43.12,47.25 42.5,47.25
N$205
  Top 0.254: 42.75,48.38 42.62,48.38 42.62,47.38
N$206
  Top 0.254: 42.88,48.25 42.75,48.25 42.75,47.5
N$207
  Top 0.254: 39.38,47.38 39.38,48.38
N$208
  Top 0.254: 43,48.38 42.88,48.38 42.88,47.38
N$209
  Top 0.254: 39.12,45.25 40.75,45.25
N$210
  Top 0.254: 39.38,44 40.38,44 40.38,45 | 40.38,45 40.38,45.12 | 40.38,45 39.5,45
N$211
  Top 0.254: 39.5,44.88 40.25,44.88
N$212
  Top 0.254: 39.38,44.5 40.25,44.5 40.25,44.38
N$213
  Top 0.254: 39.5,44.25 40.25,44.25
N$214
  Top 0.254: 36.5,45.25 36,45.25 36,44 36.5,44
N$215
  Top 0.254: 36.12,45.12 36.12,44.12
N$216
  Top 0.254: 36.25,45.12 36.25,44.25
N$217
  Top 0.254: 44,47.38 45,47.38 45,47.5
N$218
  Top 0.254: 43.88,51.25 43.88,51.75
N$219
  Top 0.254: 44.12,51.75 44,51.75 44,51.38
N$220
  Top 0.254: 45.12,51.38 45.12,51.5 | 45.12,51.5 45.12,51.62 | 45.12,51.62 45.12,51.75 | 45.12,51.5 44.12,51.5 | 45.12,51.62 44.38,51.62
N$221  (via drill 0.6 pad 1.68)
  other vias: 22.12,46.88
N$222  (via drill 0.6 pad 1.68)
  other vias: 21.75,42.88
N$223  (1 unrouted)
  Top 0.254: 19.5,47.88 18.75,47.88 18.75,49.5 19,49.5 | 9.25,55.38 8.62,55.38 | 8.62,55.38 8.62,54.75 | 8,54.12 9.12,54.12 | 8.62,55.38 8.25,55.38 8.25,54.25 8.5,54.25 | 20.5,48.88 20.5,49.5 19.25,49.5 19,49.5 | 19,49.5 19,48 19.12,48 19.12,48.38
  Top 0.305: Q1.2 16.25,50.62 | 11,40.62 11.02,40.64 | 8,54.12 8.62,54.75 C2.1 | R1.1 19.25,48.95 19.25,49.5 19.25,49.75 19.12,49.88
  Top 0.61: 11,40.62 8,40.62 8,54.12 | 17,50.62 17,54.45 | Q1.2 17,50.62 | 19.12,49.88 17,49.88 17,50.62
N$224  (via drill 0.7 pad 1.68)
  Top 0.305: 11,43.25 v11.75,43.25
  Top 0.406: 9.75,44.5 11,43.25
N$225
  Top 0.305: 14.25,43.12 14.12,43 13.38,43 12.38,42 9.75,42
N$226  (via drill 0.6 pad 1.27)
  other vias: 9.38,43
N$227  (via drill 0.6 pad 1.27)
  other vias: 9.38,45.62
N$228  (via drill 0.6 pad 1.27)
  other vias: 9.12,47.5
N$229  (via drill 0.6 pad 1.27)
  other vias: 10.12,47.5
N$230
  Top 0.305: 13.38,54.62 13.38,54.5
  Top 0.406: 10.62,47.5 11.62,47.5 12.38,48.25 13.38,48.25
  Top 0.61: 13.38,48.25 13.38,54.5
N$231
  Top 0.305: U1.47 39.12,40.25 43.38,44.5 46.38,44.5 JP4.15 | U$2.2 47.62,48.3 | 47.62,45.75 JP4.15 | JP4.15
  Top 0.61: 47.62,48.3 47.62,45.75
N$232
  Top 0.305: 23.38,46.38 23.75,46.75 24.38,46.12 24.38,46 23.88,46.5 23.75,46.5 23.38,46.12 23.75,45.75 24,46 24.12,46 23.88,46.25 23.75,46.25 23.75,46
N$233
  Top 0.305: 23.38,27.62 23.88,27.12 24.62,27.88 | 24.62,27.88 24.75,28 24.5,28.25 23.88,27.62 23.62,27.62 23.88,27.38 24.38,27.88 24.62,27.88
N$234
  Top 0.305: 22.62,26.5 21.75,25.62 22.75,24.62
N$235
  Top 0.305: 22,25.75 22.75,25 22.75,24.88
N$236
  Top 0.305: 23,25 23,25.12
N$237
  Top 0.305: 24,26.88 24.88,27.75 24.88,27.88 24,27 24,26.88 | 24,26.88 23.38,27.5
N$238
  Top 0.305: 27.62,38.5 27.62,37.75 27.5,37.88 27.5,40
N$239
  Top 0.305: 32.38,40.38 32.5,40.25 33,40.25
N$240
  Top 0.305: 27.12,40.12 27.12,39.5 27.25,39.62 27.25,40 27.38,39.88 28.88,39.88 28.88,39.62 | 28.88,39.62 28.88,39.5 27.62,39.5 27.62,39.75 27.75,39.62 28.88,39.62

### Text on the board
Top: 1 | STM32F405 | OK1FVV | CANSAT2012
